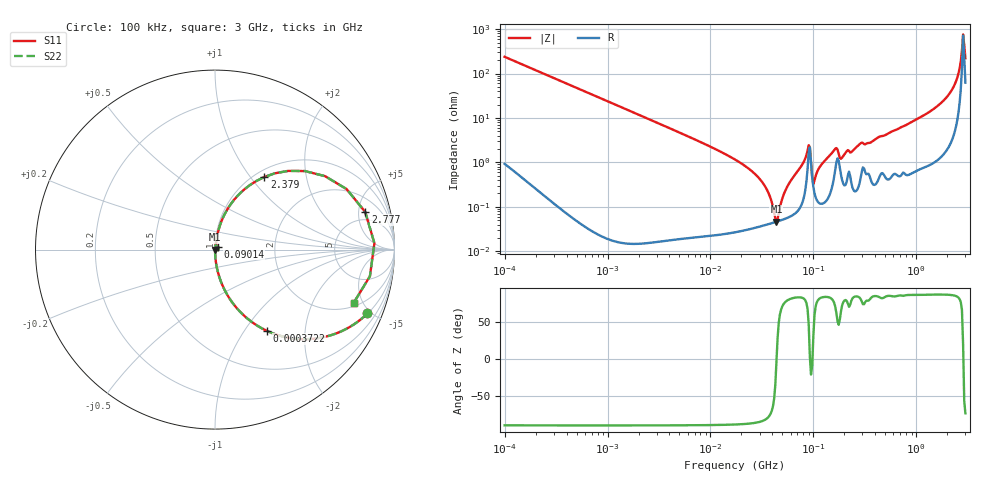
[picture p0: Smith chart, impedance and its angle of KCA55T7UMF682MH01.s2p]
!Murata Part Number: KCA55T7UMF682MH01
!These Parameters are Measured in Series Mode Connection
!Data Generated on Jan 08, 2026
!  o--ll--o
!Port1  Port2
!  o------o
!Operation Temp=25[degC], DC Bias Voltage=0[V]
!Freq. Start=100[kHz] Stop=3[GHz] 401[Steps]
# Hz S RI R 50
!Freq.(Hz) S11(Real) S11(Imag) S21(Real) S21(Imag) S12(Real) S12(Imag) S22(Real) S22(Imag)
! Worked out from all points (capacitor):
!   401 points, 100 kHz to 3 GHz, reference 50 ohm
!   read as one part in series: C = 6.67 nF near 105.3 kHz
!   lowest |Z| = 46.4 mohm at 43.8 MHz (marker M1)
!   series resonance near 43.93 MHz, so ESL is about 2 nH
!   S11 on the Smith chart (normalised r, x): 100 kHz: 1.02, -4.77; 372.2 kHz: 1.00, -1.28; 90.14 MHz: 1.03, +0.03; 2.379 GHz: 1.10, +1.18; 2.777 GHz: 3.62, +5.94; 3 GHz: 2.25, -4.25
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100000  0.8494 -0.3558  0.1506 0.3558  0.1506 0.3558  0.8494 -0.3558
372249  0.2915 -0.4538  0.7085 0.4538  0.7085 0.4538  0.2915 -0.4538
562235  0.1528 -0.3594  0.8472 0.3594  0.8472 0.3594  0.1528 -0.3594
3161081  0.00576 -0.0746  0.9942 0.0746  0.9942 0.0746  0.00576 -0.0746
1.77727e7  0.000396 -0.0112  0.9996 0.0112  0.9996 0.0112  0.000396 -0.0112
3.215051e7  0.000387 -0.00347  0.9996 0.00347  0.9996 0.00347  0.000387 -0.00347
3.657227e7  0.000412 -0.00203  0.9996 0.00203  0.9996 0.00203  0.000412 -0.00203
4.380277e7  0.000463 -3.17e-05  0.9995 3.17e-05  0.9995 3.17e-05  0.000463 -3.17e-05
5.523785e7  0.000566 0.00267  0.9994 -0.00267  0.9994 -0.00267  0.000566 0.00267
9.013636e7  0.0171 0.0169  0.9829 -0.0169  0.9829 -0.0169  0.0171 0.0169
9.738194e7  0.00461 -0.000773  0.9954 0.000773  0.9954 0.000773  0.00461 -0.000773
1.025331e8  0.00204 0.00333  0.998 -0.00333  0.998 -0.00333  0.00204 0.00333
1.196798e8  0.00125 0.00882  0.9988 -0.00882  0.9988 -0.00882  0.00125 0.00882
1.630551e8  0.00711 0.0188  0.9929 -0.0188  0.9929 -0.0188  0.00711 0.0188
1.90323e8  0.00412 0.0121  0.9959 -0.0121  0.9959 -0.0121  0.00412 0.0121
2.874592e8  0.00504 0.0263  0.995 -0.0263  0.995 -0.0263  0.00504 0.0263
5.475153e8  0.00629 0.0458  0.9937 -0.0458  0.9937 -0.0458  0.00629 0.0458
1.701687e9  0.0522 0.1942  0.9478 -0.1942  0.9478 -0.1942  0.0522 0.1942
2.378954e9  0.2756 0.4048  0.7244 -0.4048  0.7244 -0.4048  0.2756 0.4048
2.570185e9  0.5019 0.4375  0.4981 -0.4375  0.4981 -0.4375  0.5019 0.4375
2.776789e9  0.8369 0.2096  0.1631 -0.2096  0.1631 -0.2096  0.8369 0.2096
3e9  0.7726 -0.2968  0.2274 0.2968  0.2274 0.2968  0.7726 -0.2968
